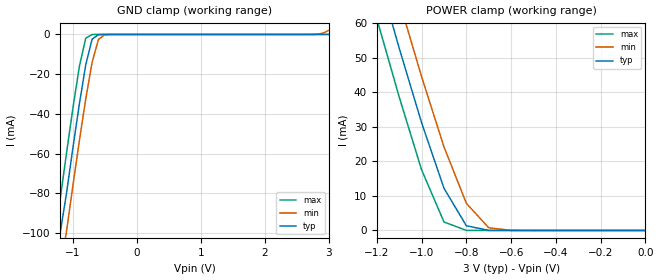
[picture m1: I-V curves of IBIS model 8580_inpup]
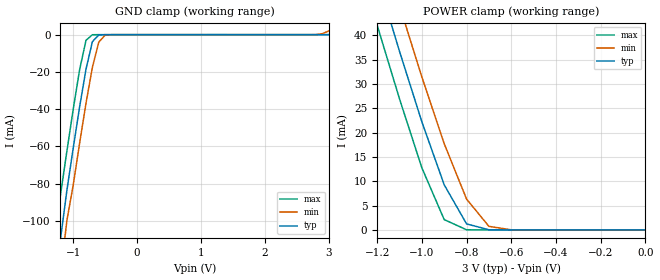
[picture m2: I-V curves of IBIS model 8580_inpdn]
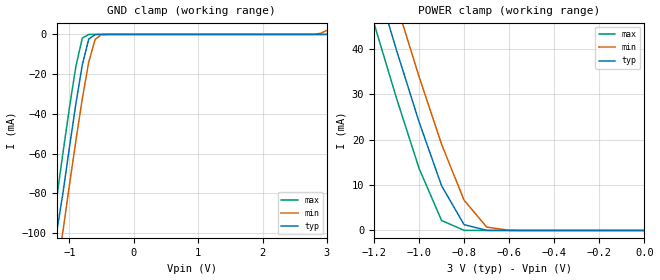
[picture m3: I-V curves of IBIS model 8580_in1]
|IBIS file 7301_3.ibs
[IBIS ver]   3.2
[File name]   7301_3.ibs
[File Rev]   3.0
[Date]   Oct 26, 2006
[Source]   This file orginated at EPSON TOYOCOM Corp.
[Copyright]   Copyright EPSON TOYOCOM Corp. 2006
|   Component RTC-7301SF
[Component]   RTC-7301SF
[Manufacturer]   EPSON TOYOCOM Corp.
[Package]
| variable   typ   min   max
R_pkg   3.00m   1.00m   5.00m
L_pkg   3.70nH   2.50nH   4.90nH
C_pkg   0.70pF   0.50pF   0.90pF
[Pin]  signal_name   model_name   R_pin   L_pin   C_pin
1   CS0N   8580_inpup
2   FCON   8580_in1
3   FOUT   8580_3state
|4   VTEMP
|5   (VDD)
6   IRQN   8580_od
7   A0   8580_in3
8   A1   8580_in3
9   A2   8580_in3
10   A3   8580_in3
11   RDN   8580_in2
12   VSS   GND
13   WRN   8580_in2
14   D3   8580_io
15   D2   8580_io
16   D1   8580_io
17   D0   8580_io
18   CS1   8580_inpdn
|19   (VDD)
|20   (VDD)
|21   (VDD)
|22   (VDD)
|23   (VDD)
24   VDD   POWER
| Models and submodels in the file (8): 8580_inpup (Input), 8580_inpdn (Input), 8580_in1 (Input), 8580_in2 (Input), 8580_in3 (Input), 8580_3state (3-state), 8580_io (I/O), 8580_od (Open_drain)
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|   Model 8580_inpup
[Model]   8580_inpup
Model_type   Input
Vinl =   0.60V
Vinh =   2.40V
C_comp   8.00pF   8.00pF   8.00pF
[Temperature Range]   25.00   85.00   -40.00
[Voltage Range]   3.00V   2.40V   3.60V
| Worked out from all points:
|   GND clamp passes 1 mA (typ) near -0.64 V on its own axis
|   POWER clamp passes 1 mA (typ) near -0.77 V on its own axis
[GND_clamp]
| voltage   I(typ)   I(min)   I(max)
-3V       -540mA     -560mA     -520mA
-1.3V     -130mA     -150mA     -110mA
-1.2V     -100mA     -120mA     -82.93mA
-1.1V     -79.75mA   -98.87mA   -59.59mA
-1V       -56.92mA   -75.91mA   -36.99mA
-900mV    -35.03mA   -53.6mA    -16.15mA
-800mV    -15.34mA   -32.47mA   -1.91mA
-700mV    -2.37mA    -13.97mA   -39.59uA
-600mV    -78.87uA   -2.44mA    -20.77uA
-500mV    -11.62uA   -130uA     -20.65uA
2.8V      -2.04uA    42.04uA    -11.74uA
3V        3.08pA     2.01mA     -9.27uA
[POWER_clamp]
| voltage   I(typ)   I(min)   I(max)
-3V       510mA      530mA      500mA
-1.2V     75.5mA     89.14mA    61.27mA
-1.1V     52.76mA    66.39mA    38.61mA
-1V       31.18mA    44.5mA     17.55mA
-900mV    12.21mA    24.18mA    2.45mA
-800mV    1.35mA     7.85mA     27.44uA
-700mV    33.84uA    770uA      190nA
-600mV    690nA      33.31uA    1.31nA
0V        3pA        14.46pA    3.6pA
|   Model 8580_inpdn
[Model]   8580_inpdn
Model_type   Input
Vinl =   0.60V
Vinh =   2.40V
C_comp   8.00pF   8.00pF   8.00pF
[Temperature Range]   25.00   85.00   -40.00
[Voltage Range]   3.00V   2.40V   3.60V
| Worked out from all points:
|   GND clamp passes 1 mA (typ) near -0.62 V on its own axis
|   POWER clamp passes 1 mA (typ) near -0.78 V on its own axis
[GND_clamp]
| voltage   I(typ)   I(min)   I(max)
-3V       -550mA     -570mA     -530mA
-1.3V     -130mA     -150mA     -110mA
-1.2V     -110mA     -130mA     -86.2mA
-1.1V     -83.87mA   -100mA     -62.79mA
-1V       -60.92mA   -80.78mA   -40.05mA
-900mV    -38.82mA   -58.3mA    -18.83mA
-800mV    -18.56mA   -36.84mA   -3.02mA
-700mV    -3.78mA    -17.56mA   -37.75uA
-600mV    -140uA     -3.99mA    -260nA
-500mV    -2.83uA    -250uA     -1.81nA
2.8V      4.5uA      40.88uA    10.29uA
3V        4.5uA      2mA        10.3uA
[POWER_clamp]
| voltage   I(typ)   I(min)   I(max)
-3V       340mA      350mA      340mA
-1.2V     51.94mA    61.35mA    42.11mA
-1.1V     36.73mA    46.14mA    26.96mA
-1V       22.24mA    31.45mA    12.78mA
-900mV    9.28mA     17.73mA    2.13mA
-800mV    1.25mA     6.35mA     37.67uA
-700mV    38.25uA    740uA      10.49uA
-600mV    5.19uA     35.14uA    10.3uA
0V        4.5uA      1.9uA      10.3uA
|   Model 8580_in1
[Model]   8580_in1
Model_type   Input
Vinl =   0.60V
Vinh =   2.40V
C_comp   8.00pF   8.00pF   8.00pF
[Temperature Range]   25.00   85.00   -40.00
[Voltage Range]   3.00V   2.40V   3.60V
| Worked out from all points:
|   GND clamp passes 1 mA (typ) near -0.64 V on its own axis
|   POWER clamp passes 1 mA (typ) near -0.78 V on its own axis
[GND_clamp]
| voltage   I(typ)   I(min)   I(max)
-3V       -540mA     -560mA     -520mA
-1.3V     -130mA     -150mA     -110mA
-1.2V     -100mA     -120mA     -82.91mA
-1.1V     -79.74mA   -98.87mA   -59.57mA
-1V       -56.91mA   -75.91mA   -36.97mA
-900mV    -35.02mA   -53.6mA    -16.13mA
-800mV    -15.33mA   -32.47mA   -1.89mA
-700mV    -2.36mA    -13.97mA   -18.95uA
-600mV    -68.66uA   -2.44mA    -130nA
-500mV    -1.41uA    -130uA     -910pA
2.8V      2.64pA     38.98uA    2pA
3V        3.08pA     2mA        2.4pA
[POWER_clamp]
| voltage   I(typ)   I(min)   I(max)
-3V       370mA      380mA      370mA
-1.2V     56.28mA    66.47mA    45.64mA
-1.1V     39.7mA     49.89mA    29.11mA
-1V       23.92mA    33.89mA    13.68mA
-900mV    9.84mA     18.96mA    2.19mA
-800mV    1.27mA     6.66mA     27.39uA
-700mV    33.78uA    750uA      190nA
-600mV    690nA      33.26uA    1.31nA
0V        3pA        14.46pA    3.6pA
